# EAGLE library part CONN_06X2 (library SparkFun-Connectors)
Multi connection point. Often used as Generic Header-pin footprint for 0.1 inch spaced/style header connections On any of the 0.1 inch spaced packages, you can populate with these: Break Away Headers - Straight (PRT-00116) Break Away Male Headers - Right Angle (PRT-00553) Female Headers (PRT-00115) Break Away Headers - Machine Pin (PRT-00117) Break Away Female Headers - Swiss Machine Pin (PRT-00743)
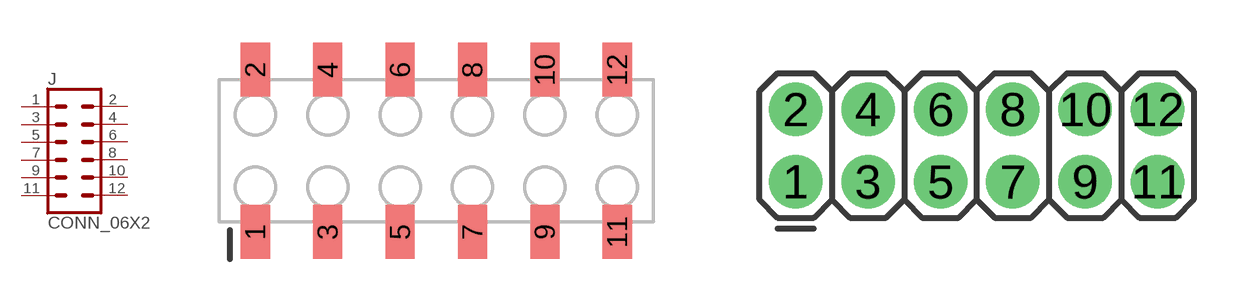
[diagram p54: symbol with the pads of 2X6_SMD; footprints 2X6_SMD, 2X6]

Designator prefix J

## CONN_06X2SMD_FEMALE  [2X6_SMD]
1  1  pas
2  2  pas
3  3  pas
4  4  pas
5  5  pas
6  6  pas
7  7  pas
8  8  pas
9  9  pas
10  10  pas
11  11  pas
12  12  pas

## CONN_06X2PTH_FEMALE (PROD_ID: CONN-12423; VALUE: 2X6 FEMALE)  [2X6]
Pads as for 2X6_SMD

## CONN_06X2NO_SILK  [2X6_NOSILK]
Pads as for 2X6_SMD

## Footprint 2X6_SMD (pad centres in mm)
Surface Mount - 2x6 Specifications: Pin count:12 Pin pitch:0.1" Example device(s): CONN_06x2
smd 1.02 x 1.9: 1 -6.35,-2.85; 2 -6.35,2.85; 3 -3.81,-2.85; 4 -3.81,2.85; 5 -1.27,-2.85; 6 -1.27,2.85; 7 1.27,-2.85; 8 1.27,2.85; 9 3.81,-2.85; 10 3.81,2.85; 11 6.35,-2.85; 12 6.35,2.85

## Footprint 2X6 (pad centres in mm)
Plated Through Hole - 2x6 Specifications: Pin count:12 Pin pitch:0.1" Example device(s): CONN_06x2
drill 1.016 pad 1.88: 1 0,0; 2 0,2.54; 3 2.54,0; 4 2.54,2.54; 5 5.08,0; 6 5.08,2.54; 7 7.62,0; 8 7.62,2.54; 9 10.16,0; 10 10.16,2.54; 11 12.7,0; 12 12.7,2.54

## Footprint 2X6_NOSILK (pad centres in mm)
drill 1.016 pad 1.88: 1 0,0; 2 0,2.54; 3 2.54,0; 4 2.54,2.54; 5 5.08,0; 6 5.08,2.54; 7 7.62,0; 8 7.62,2.54; 9 10.16,0; 10 10.16,2.54; 11 12.7,0; 12 12.7,2.54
